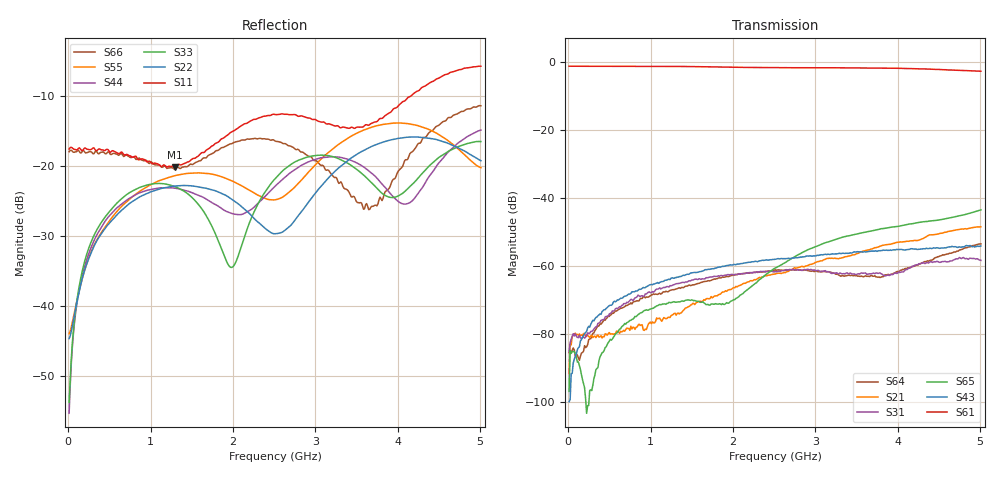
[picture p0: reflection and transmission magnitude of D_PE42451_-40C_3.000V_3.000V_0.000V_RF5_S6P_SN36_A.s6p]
! Device ID: PE42451
! Serial: 36
! Insertion: A
! Temp: -40C
! VDD: 3.000
! Control_Hi: 100.000
! Control_Lo: 0.000
! Logic State: RF5
! Port 1: RFC
! Port 2: RF1
! Port 3: RF2
! Port 4: RF3
! Port 5: RF4
! Port 6: RF5
! V1 = 3.00
! V2 = 0.00
! V3 = 3.00
! V4 = 0.00
! IDD: 1.322070e-05
#  Hz  S  RI  R  50
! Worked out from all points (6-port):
!   401 points, 10 MHz to 5.01 GHz, reference 50 ohm
!   strongest paths, dB at 10 MHz, 1.26 GHz, 2.51 GHz, 3.76 GHz, 5.01 GHz:
!     S61: -1.3, -1.4, -1.8, -1.9, -2.8
!     S43: -99.8, -63.4, -58.0, -55.6, -54.1
!     S65: -96.8, -70.6, -60.6, -49.3, -43.5
!     S31: -85.1, -65.7, -61.6, -62.1, -58.3
!     S21: -91.5, -74.4, -62.3, -54.4, -48.5
!     S64: -85.4, -67.0, -61.0, -63.3, -53.5
!   lowest |S11| = -20.2 dB at 1.298 GHz (marker M1), VSWR 1.22, Z = 54 - j9.43 ohm
!   |S11| at or under -10 dB: start of sweep to 4.161 GHz
